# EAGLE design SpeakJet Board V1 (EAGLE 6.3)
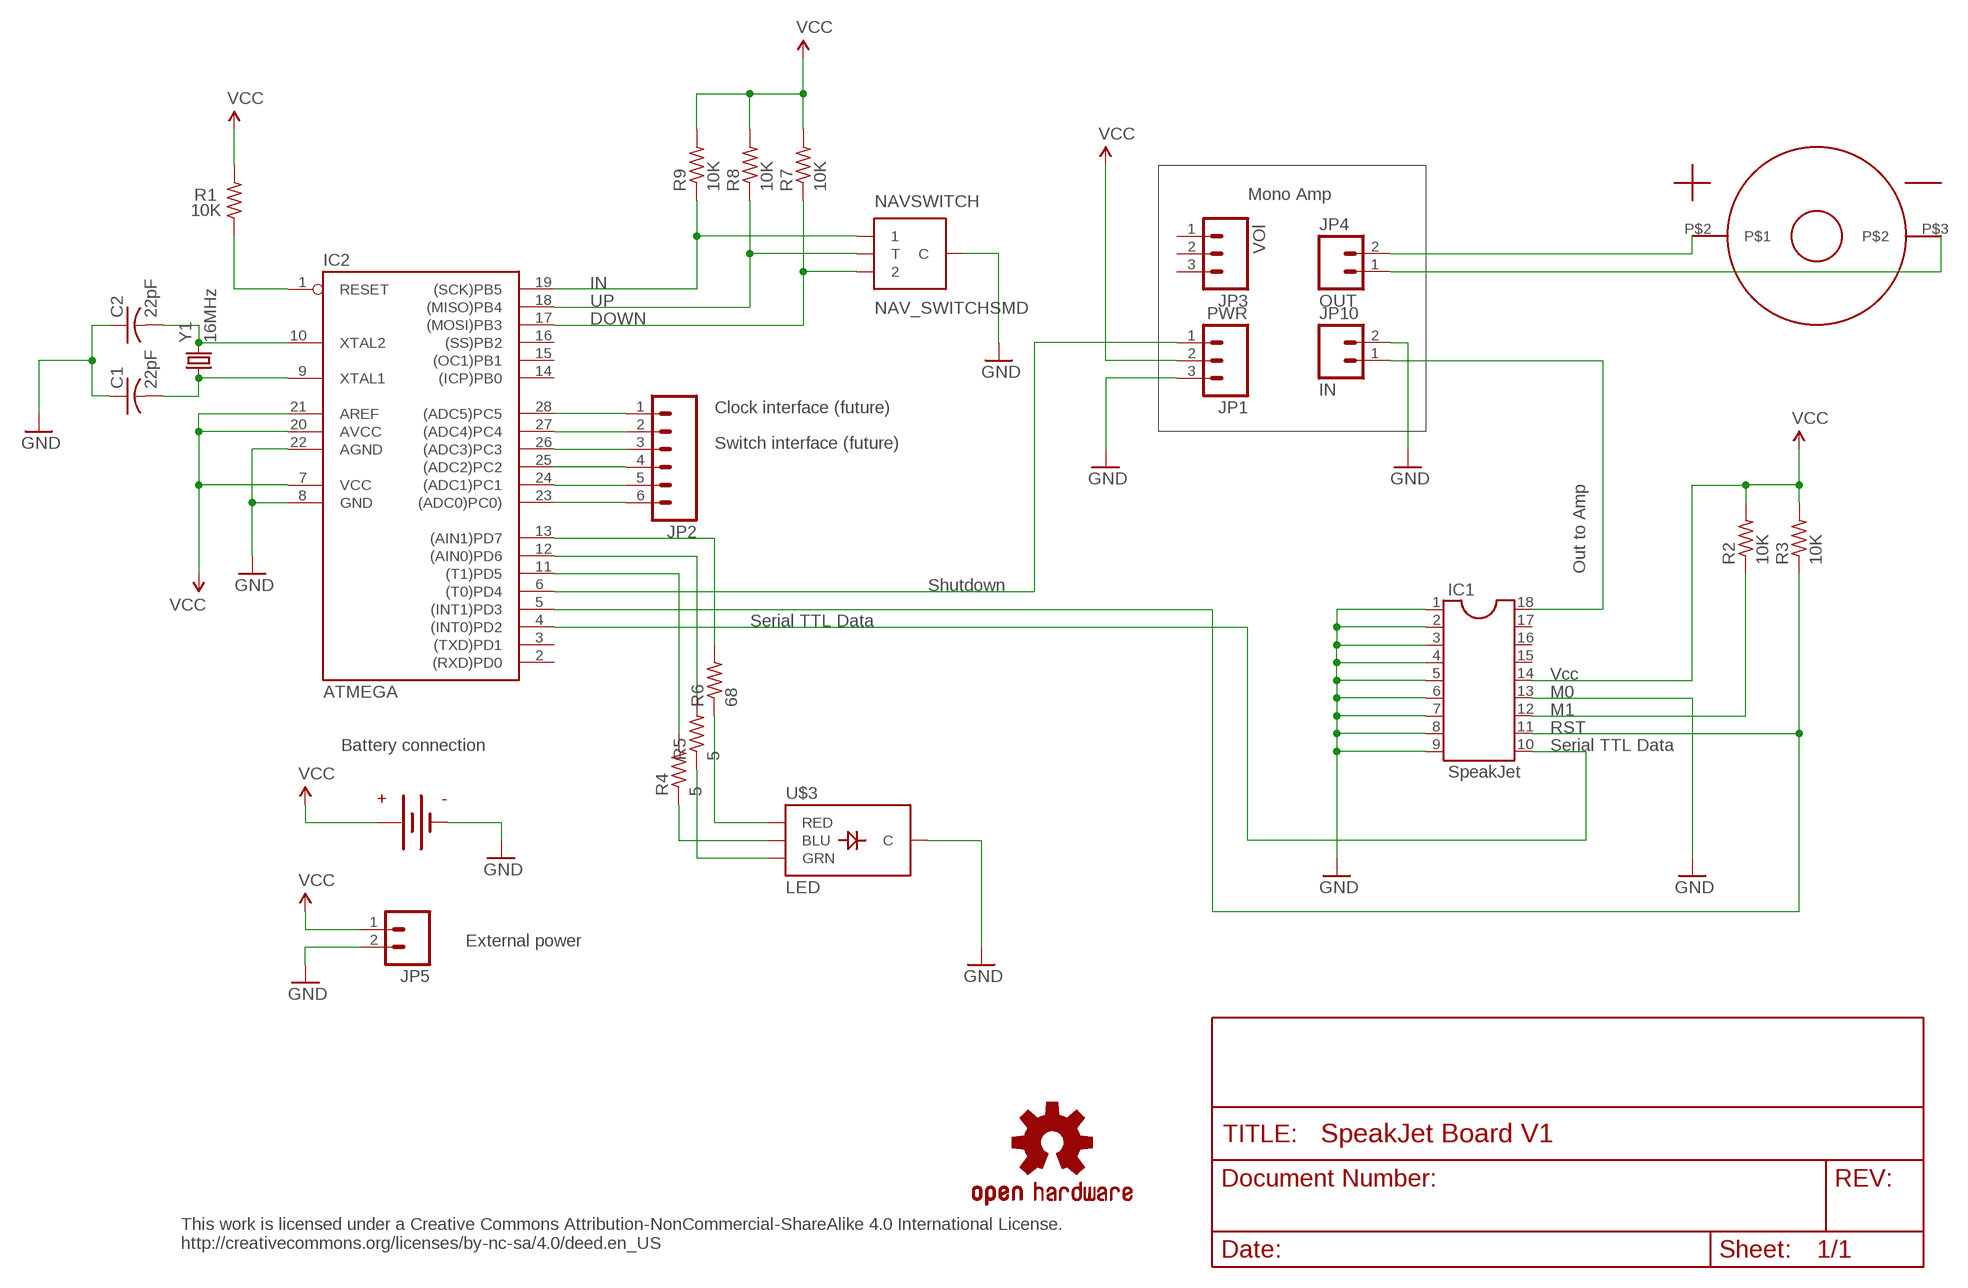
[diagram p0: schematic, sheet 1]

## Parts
C1  22pF  C-USC0805  [C0805]
C2  22pF  C-USC0805  [C0805]
IC1  SpeakJet  DIL18  [DIL18]
IC2  ATMEGA  AT90S4433P  [DIL28-3]
JP1  PWR  M03PTH  [1X03]
JP2  M06SIP  [1X06]
JP3  M03PTH  [1X03]
JP4  OUT  M02PTH  [1X02]
JP5  M02PTH  [1X02]
JP10  IN  M02PTH  [1X02]
NAVSWITCH  NAV_SWITCHSMD  [NAV_SWITCH]
R1  10K  R-US_M0805  [M0805]
R2  10K  R-US_M0805  [M0805]
R3  10K  R-US_M0805  [M0805]
R4  5  R-US_M0805  [M0805]
R5  5  R-US_M0805  [M0805]
R6  68  R-US_M0805  [M0805]
R7  10K  R-US_M0805  [M0805]
R8  10K  R-US_M0805  [M0805]
R9  10K  R-US_M0805  [M0805]
U$1  OSHW-LOGOS  [OSHW-LOGO-S]
U$3  LED  LED-TRICOLOR-THROUGHHOLE  [LED-TRICOLOR-THROUGHHOLE]
U$4  SPEAKER_WITH_PADS_28MM  [SPEAKER_WITH_PAD_28MM]
U$5  1-2AA_BATTERY_HOLDER  [1/2AA_BATTERY_HOLDER_BH1]
Y1  16MHz  CRYSTAL5X3  [CRYSTAL-SMD-5X3]

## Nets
GND [power]: C1.1 C2.1 IC1.1 IC1.2 IC1.3 IC1.4 IC1.5 IC1.6 IC1.7 IC1.8 IC1.9 IC1.13 IC2.8(GND) IC2.22(AGND) JP1.3 JP5.2 JP10.2 NAVSWITCH.C U$3.GND(C) U$5.P$1(-)
N$1 [power]: IC1.18 JP10.1
N$2: IC2.6((T0)PD4) JP1.1
N$3: JP4.2 U$4.P$2
N$4: JP4.1 U$4.P$3
N$5: IC2.18((MISO)PB4) NAVSWITCH.T R8.1
N$6: IC2.19((SCK)PB5) NAVSWITCH.1 R9.1
N$7: IC2.13((AIN1)PD7) R6.2
N$8: C1.2 IC2.9(XTAL1) Y1.1
N$9: C2.2 IC2.10(XTAL2) Y1.3
N$10: IC2.17((MOSI)PB3) NAVSWITCH.2 R7.1
N$11: IC2.1(RESET) R1.1
N$12: IC1.12 R2.1
N$13: IC1.11 IC2.5((INT1)PD3) R3.1
N$14: IC2.12((AIN0)PD6) R5.2
N$15: IC2.11((T1)PD5) R4.2
N$16: IC1.10 IC2.4((INT0)PD2)
N$18: IC2.28((ADC5)PC5) JP2.1
N$19: IC2.27((ADC4)PC4) JP2.2
N$20: IC2.26((ADC3)PC3) JP2.3
N$21: IC2.25((ADC2)PC2) JP2.4
N$22: IC2.24((ADC1)PC1) JP2.5
N$23: IC2.23((ADC0)PC0)) JP2.6
N$24: R4.1 U$3.BLU
N$25: R5.1 U$3.GRN
N$26: R6.1 U$3.RED
VCC: IC1.14 IC2.7(VCC) IC2.20(AVCC) IC2.21(AREF) JP1.2 JP5.1 R1.2 R2.2 R3.2 R7.2 R8.2 R9.2 U$5.P$2(+)
Unconnected: IC1.15 IC1.16 IC1.17 IC2.2((RXD)PD0) IC2.3((TXD)PD1) IC2.14((ICP)PB0) IC2.15((OC1)PB1) IC2.16((SS)PB2) JP3.1 JP3.2 JP3.3

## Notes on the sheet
- Mono Amp
- VOl
- IN
- UP
- DOWN
- Clock interface (future)
- Switch interface (future)
- Out to Amp
- Shutdown
- Serial TTL Data
- Vcc
- M0
- M1
- RST
- Battery connection | Serial TTL Data
- External power
- This work is licensed under a Creative Commons Attribution-NonCommercial-ShareAlike 4.0 International License.
  http://creativecommons.org/licenses/by-nc-sa/4.0/deed.en_US

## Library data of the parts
C1 C2 = adafruit:C-US: CAPACITOR, American symbol
IC1 = ic-package:DIL18: Dual In Line / Socket
IC2 = atmel:AT90S4433: MICROCONTROLLER 4 Kbytes FLASH 128 bytes SRAM 256 bytes EEPROM UART 6-channel 10 bit ADC
JP1 JP3 = SparkFun:M03: Header 3 Standard 3-pin 0.1" header. Use with straight break away headers (SKU : PRT-00116), right angle break away headers (PRT-00553), swiss pins (PRT-00743), machine pins (PRT-00117), and female headers (PRT-00115). Molex polarized connector foot print use with SKU : PRT-08232 with associated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
JP2 = SparkFun:M06: Header 6 Standard 6-pin 0.1" header. Use with straight break away headers (SKU : PRT-00116), right angle break away headers (PRT-00553), swiss pins (PRT-00743), machine pins (PRT-00117), and female headers (PRT-00115). Molex polarized connector foot print use with SKU : PRT-08094 with associated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
JP4 JP5 JP10 = SparkFun:M02: Header 2
NAVSWITCH = SparkFun:NAV_SWITCH: Navigation Switch Three way navigation switch. Commonly used as up/down/select on MP3 players. Schematic element and footprint production proven. Spark Fun Electronics SKU : COM-08184
R1-R9 = adafruit:R-US_: RESISTOR, American symbol
U$1 = SparkFun:OSHW-LOGO: Open Source Hardware Logo This logo indicates the piece of hardware it is found on incorporates a OSHW license and/or adheres to the definition of open source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
U$3 = SparkFun w:epaper:LED-TRICOLOR-THROUGHHOLE
U$4 = Speaker with pad:SPEAKER_WITH_PADS_28MM: SPEAKER 8 OHM .25W 28MM ROUND
U$5 = 1-2AA battery holder:1-2AA_BATTERY_HOLDER: Battery holder for 1/2AA 3.6V cells
Y1 = SparkFun-FreqCtrl:CRYSTAL: Various standard crystals. Proven footprints. Spark Fun Electronics SKU : COM-00534

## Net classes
1 power: width 0.6 mm, clearance 0.3 mm

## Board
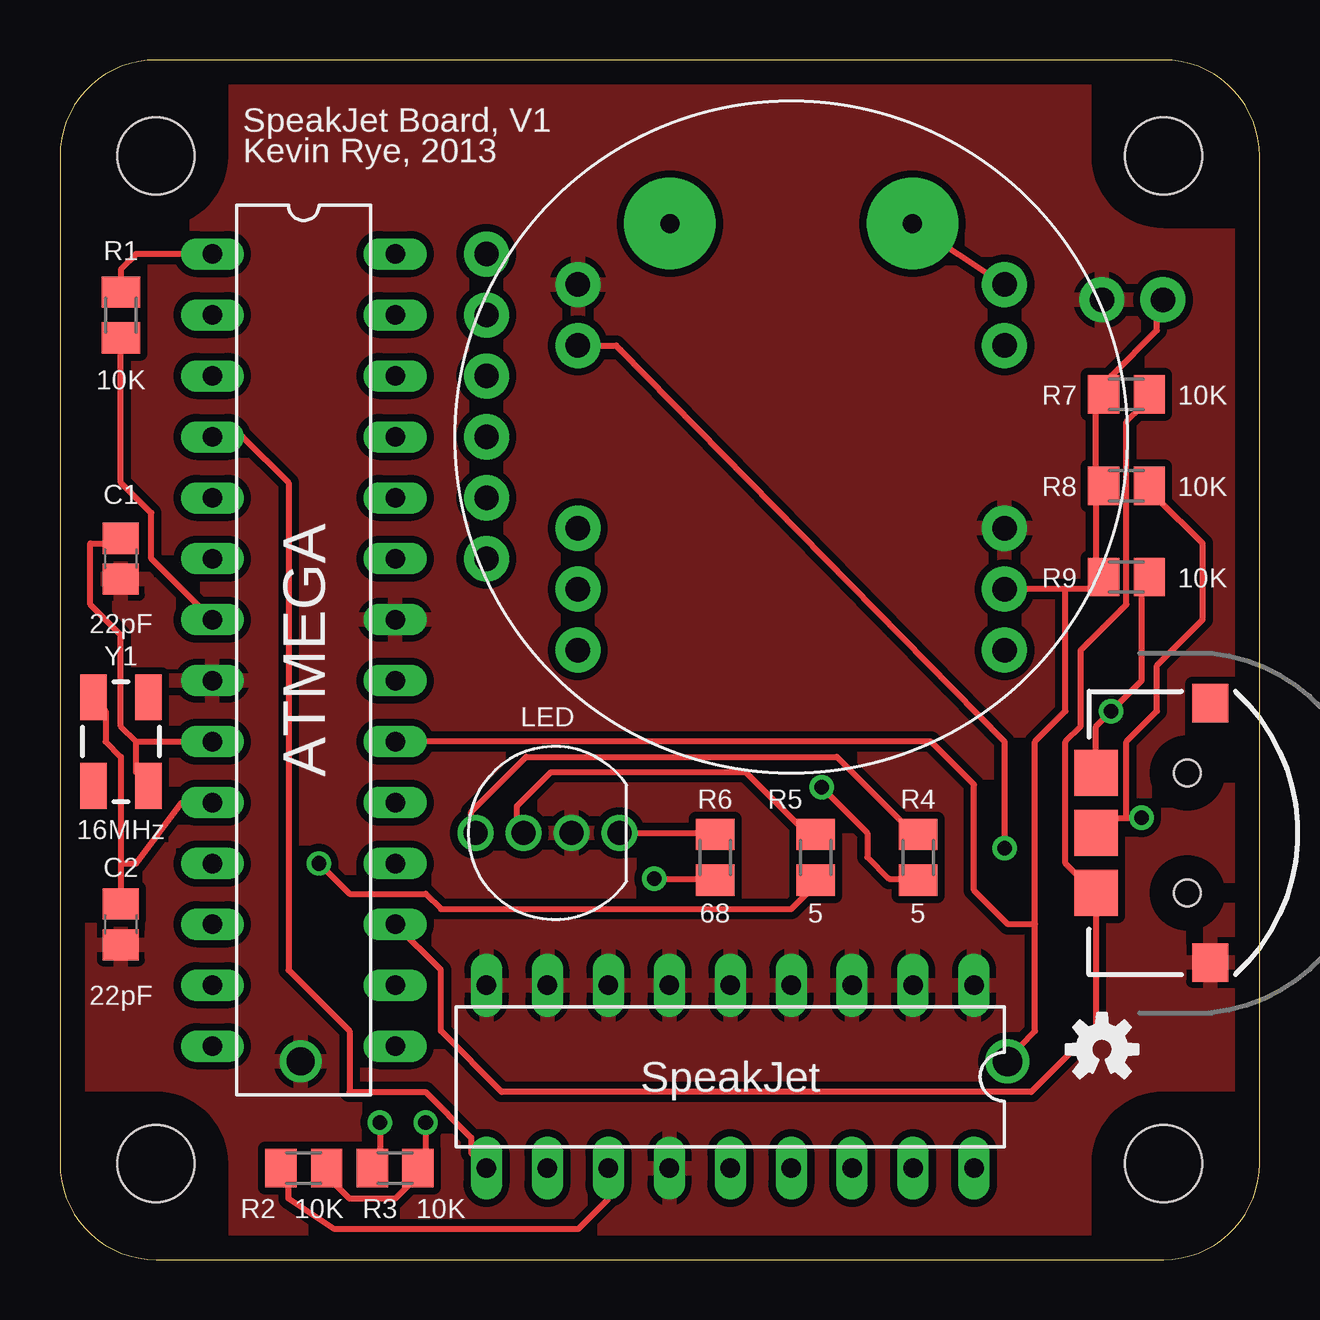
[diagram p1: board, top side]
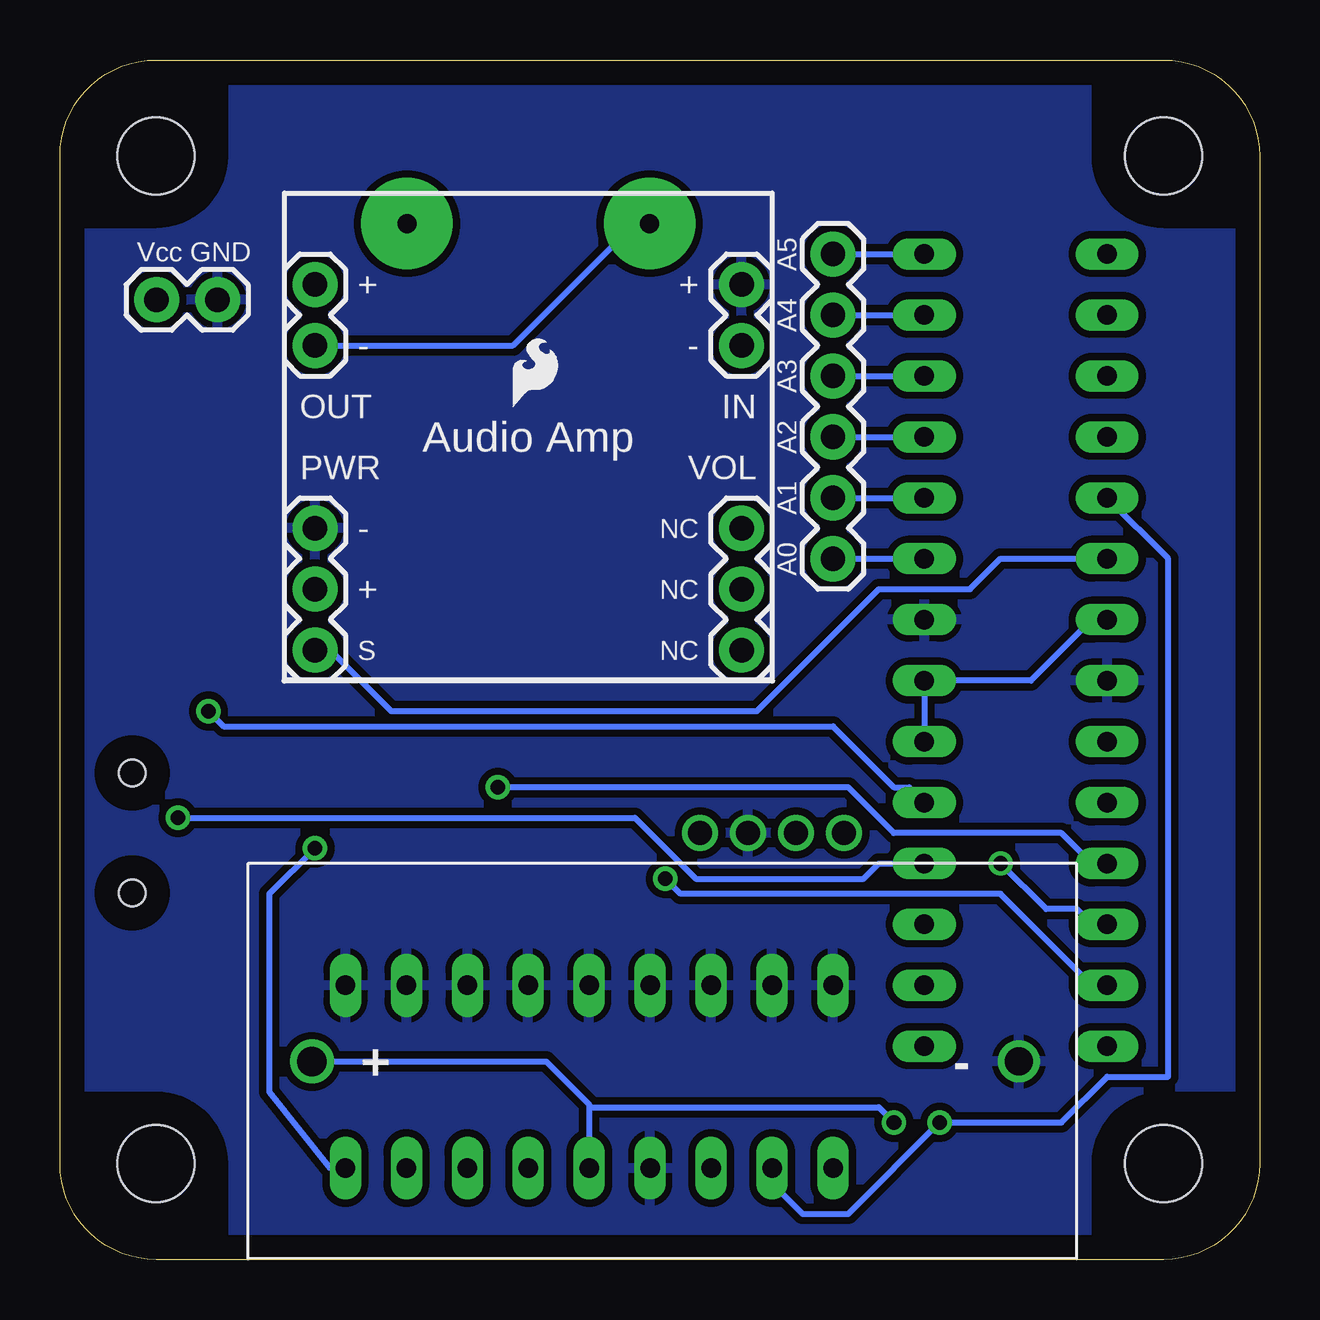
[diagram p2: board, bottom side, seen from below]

Size 50 x 50 mm. Coordinates in mm from the lower left corner, seen from the top.
Copper layers (1*16): Top 0.035mm / dielectric 1.5mm / Bottom 0.035mm
Design rules "default": minimum track width 10mil, minimum drill 24mil, track to track 8mil, track to pad 8mil, pad to pad 8mil, via to via 8mil, smd to smd 8mil, copper to edge 40mil, drill to drill 8mil, minimum pad ring 10mil, minimum via ring 8mil, stop-mask expansion 4mil, vias tented up to drill 0mil, thermal gap 10mil

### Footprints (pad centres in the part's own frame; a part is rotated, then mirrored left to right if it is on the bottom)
C0805 = smd 1.3 x 1.5: 1 -0.85,0; 2 0.85,0
DIL18 = drill 0.813 long: 1 -10.16,-3.81; 2 -7.62,-3.81; 3 -5.08,-3.81; 4 -2.54,-3.81; 5 0,-3.81; 6 2.54,-3.81; 7 5.08,-3.81; 8 7.62,-3.81; 9 10.16,-3.81; 10 10.16,3.81; 11 7.62,3.81; 12 5.08,3.81; 13 2.54,3.81; 14 0,3.81; 15 -2.54,3.81; 16 -5.08,3.81; 17 -7.62,3.81; 18 -10.16,3.81
DIL28-3 = drill 0.813 long: 1 -16.51,-3.81; 2 -13.97,-3.81; 3 -11.43,-3.81; 4 -8.89,-3.81; 5 -6.35,-3.81; 6 -3.81,-3.81; 7 -1.27,-3.81; 8 1.27,-3.81; 9 3.81,-3.81; 10 6.35,-3.81; 11 8.89,-3.81; 12 11.43,-3.81; 13 13.97,-3.81; 14 16.51,-3.81; 15 16.51,3.81; 16 13.97,3.81; 17 11.43,3.81; 18 8.89,3.81; 19 6.35,3.81; 20 3.81,3.81; 21 1.27,3.81; 22 -1.27,3.81; 23 -3.81,3.81; 24 -6.35,3.81; 25 -8.89,3.81; 26 -11.43,3.81; 27 -13.97,3.81; 28 -16.51,3.81
1X03 = drill 1.016 pad 1.88: 1 0,0; 2 2.54,0; 3 5.08,0
1X06 = drill 1.016 pad 1.88: 1 0,0; 2 2.54,0; 3 5.08,0; 4 7.62,0; 5 10.16,0; 6 12.7,0
1X02 = drill 1.016 pad 1.88: 1 0,0; 2 2.54,0
NAV_SWITCH = smd 1.9 x 1.8: 1 -2.5,-3.8; 2 2.5,-3.8; T 0,-3.8 | smd 1.6 x 1.5: C 5.4,0.95; NC -5.4,0.95 | hole 1.1: -2.5,0; 2.5,0
M0805 = smd 1.3 x 1.6: 1 -0.95,0; 2 0.95,0
DP5050_V1 = hole 3.2: 4,4; 46,4; 46,46; 4,46
LED-TRICOLOR-THROUGHHOLE = drill 1: BLU 3,0; GND -1,0; GRN 1,0; RED -3,0
SPEAKER_WITH_PAD_28MM = drill 0.8 pad 3.81: P$2 5.055,8.89; P$3 -5.055,8.89
1/2AA_BATTERY_HOLDER_BH1 = drill 1.168: P$1 2.413,8.255 | drill 1.219: P$2 31.877,8.255
CRYSTAL-SMD-5X3 = smd 1.9 x 1.1: 1 -1.85,-1.15; 2 1.85,-1.15; 3 1.85,1.15; 4 -1.85,1.15

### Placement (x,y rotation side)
C1  2.54,29.21 90 top
C2  2.54,13.97 90 top
IC1  27.94,7.62 180 top
IC2  10.16,25.4 270 top
JP1  39.37,25.4 90 bottom
JP2  17.78,41.91 270 bottom
JP3  21.59,25.4 90 bottom
JP4  39.37,38.1 90 bottom
JP5  45.97,40.01 0 bottom
JP10  21.59,38.1 90 bottom
NAVSWITCH  46.99,17.78 270 top
R1  2.54,39.37 270 top
R2  10.16,3.81 0 top
R3  13.97,3.81 0 top
R4  35.76,16.76 270 top
R5  31.5,16.76 270 top
R6  27.3,16.76 270 top
R7  44.45,36.07 180 top
R8  44.45,32.26 180 top
R9  44.45,28.45 180 top
U$1  43.43,8.76 0 top
U$2  [DP5050_V1]  0,0 0 top
U$3  20.32,17.78 180 top
U$4  30.48,34.29 0 top
U$5  7.62,16.51 180 bottom
U$7  [SFE-LOGO-FLAME]  31.11,35.56 0 bottom
Y1  2.54,21.59 90 top

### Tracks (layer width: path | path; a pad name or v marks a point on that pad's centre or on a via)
GND
  pour Bottom: -6.35,53.34 55.88,53.34 55.88,-5.08 -6.35,-5.08
  pour Top: -6.35,53.34 55.88,53.34 55.88,-5.08 -6.35,-5.08
N$1  (via drill 0.61)
  Top 0.254: v39.37,17.14 39.37,21.59 23.37,37.91 23.18,38.1 JP10.1
  Bottom 0.254: IC1.18 38.73,3.81 41.27,6.99 41.27,15.24 v39.37,17.14
N$2
  Bottom 0.254: IC2.6 10.79,29.21 12.06,27.94 15.88,27.94 20.95,22.86 36.2,22.86 38.73,25.4 JP1.1
N$3
  Top 0.254: U$4.P$2 JP4.2
N$4
  Bottom 0.254: U$4.P$3 26.04,43.18 31.11,38.1 JP4.1
N$5  (via drill 0.61)
  Top 0.254: 44.45,18.41 44.45,21.59 45.72,22.86 45.72,24.77 47.62,26.67 47.62,29.84 45.72,31.75 R8.1 | 44.45,18.41 43.81,18.41 43.81,17.78 NAVSWITCH.T | 44.45,18.41 v45.09,18.41
  Bottom 0.254: IC2.18 15.88,16.51 16.51,15.88 23.5,15.88 26.04,18.41 v45.09,18.41
N$6  (via drill 0.61)
  Top 0.254: R9.1 45.09,27.94 45.09,24.13 v43.81,22.86 43.18,22.23 43.18,20.32 NAVSWITCH.1
  Bottom 0.254: IC2.19 14.61,19.68 15.24,19.68 17.78,22.23 43.18,22.23 v43.81,22.86
N$7  (via drill 0.61)
  Top 0.254: v24.77,15.88 27.3,15.88 R6.2
  Bottom 0.254: v24.77,15.88 24.13,15.24 10.79,15.24 6.99,11.43 IC2.13
N$8
  Top 0.254: 3.17,21.59 2.54,22.23 2.54,26.04 1.27,27.3 1.27,29.84 2.54,29.84 C1.2 | 3.17,21.59 3.17,20.32 Y1.1 | 3.17,21.59 IC2.9
N$9
  Top 0.254: 2.54,16.51 2.54,20.95 1.91,21.59 1.91,22.86 Y1.3 | 2.54,16.51 C2.2 | IC2.10 5.08,19.05 3.17,16.51 2.54,16.51
N$10
  Top 0.254: 43.18,15.24 41.91,16.51 41.91,21.59 42.55,22.23 42.55,25.4 44.45,27.3 44.45,34.92 45.09,35.56 R7.1 | IC2.17 15.88,12.06 15.88,9.53 18.41,6.99 40.49,6.99 43.18,9.68 43.18,15.24 | 43.18,15.24 NAVSWITCH.2
N$11
  Top 0.254: R1.1 2.54,41.27 3.17,41.91 IC2.1
N$12
  Top 0.254: IC1.12 22.86,2.54 21.59,1.27 11.43,1.27 9.53,2.54 9.53,3.81 R2.1
N$13  (via drill 0.61)
  Top 0.254: v13.34,5.71 13.34,3.81 R3.1
  Bottom 0.254: IC1.11 20.32,3.17 19.05,1.91 17.14,1.91 v13.34,5.71 8.26,5.71 6.35,7.62 3.81,7.62 3.81,29.21 IC2.5
N$14  (via drill 0.61)
  Top 0.254: v10.79,16.51 12.06,15.24 15.24,15.24 15.88,14.61 30.48,14.61 31.11,15.24 R5.2
  Bottom 0.254: v10.79,16.51 8.89,14.61 7.62,14.61 6.99,13.97 IC2.12
N$15  (via drill 0.61)
  Top 0.254: v31.75,19.68 33.66,17.78 33.66,16.77 34.55,15.88 35.56,15.88 R4.2
  Bottom 0.254: v31.75,19.68 17.14,19.68 15.24,17.78 8.26,17.78 6.99,16.51 IC2.11
N$16
  Top 0.254: IC1.10 17.14,4.45 17.14,5.08 15.24,6.99 12.06,6.99 12.06,9.53 9.53,12.06 9.53,32.38 7.62,34.29 IC2.4
N$18
  Bottom 0.254: JP2.1 IC2.28
N$19
  Bottom 0.254: JP2.2 IC2.27
N$20
  Bottom 0.254: JP2.3 IC2.26
N$21
  Bottom 0.254: JP2.4 IC2.25
N$22
  Bottom 0.254: JP2.5 IC2.24
N$23
  Bottom 0.254: JP2.6 IC2.23
N$24
  Top 0.254: R4.1 35.56,17.78 32.38,20.95 19.43,20.95 17.14,18.66 17.14,17.78 U$3.BLU
N$25
  Top 0.254: R5.1 31.11,17.78 28.57,20.32 20.47,20.32 19.05,18.9 19.05,17.78 U$3.GRN
N$26
  Top 0.254: U$3.RED 27.3,17.78 R6.1
VCC  (via drill 0.61)
  Top 0.254: R1.2 2.54,32.38 3.81,31.11 3.81,29.21 IC2.7 | 41.91,27.94 43.18,27.94 R9.2 43.18,28.57 43.18,31.75 R8.2 43.18,32.38 43.18,35.56 R7.2 43.81,36.2 43.81,36.83 45.72,38.73 45.72,40.01 JP5.1 | 41.91,27.94 JP1.2 | R2.2 11.43,3.81 11.43,3.17 12.06,2.54 13.97,2.54 14.61,3.17 14.61,3.81 R3.2 15.24,3.81 v15.24,5.71 | 41.91,27.94 41.91,22.86 40.64,21.59 40.64,13.97 | 40.64,13.97 40.64,9.53 40.01,8.89 40.01,8.26 U$5.P$2 | 40.64,13.97 39.52,13.97 38.1,15.39 38.1,19.79 36.3,21.59 IC2.20
  Bottom 0.254: IC2.20 IC2.21 9.53,24.13 6.99,26.67 IC2.7 | U$5.P$2 29.74,8.26 27.94,6.46 27.94,6.35 | 27.94,6.35 IC1.14 | v15.24,5.71 15.88,6.35 27.94,6.35

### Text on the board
Unrouted: This work is licensed under a Creative Commons Attribution-NonCommercial-ShareAlike 4.0 International License. / http://creativecommons.org/licenses/by-nc-sa/4.0/deed.en_US
tPlace: SpeakJet Board, V1 | Kevin Rye, 2013
bPlace: A5 | GND | Vcc | + | + | A4 | - | - | A3 | IN | OUT | A2 | Audio Amp | VOL | PWR | A1 | NC | - | A0 | NC | + | NC | S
